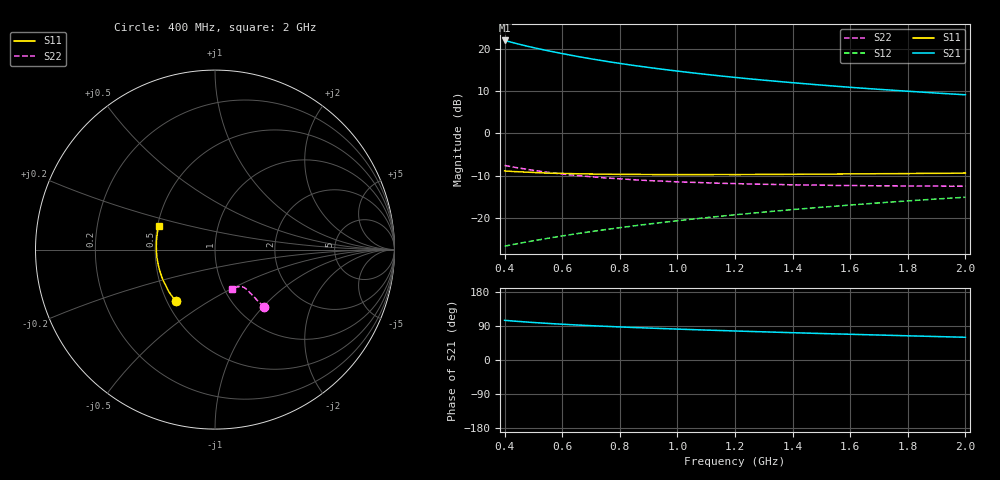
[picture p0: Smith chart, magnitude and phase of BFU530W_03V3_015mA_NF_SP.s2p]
! Filename:  P:\Prog\Test\Noise\ATS_data\Testdata_Net\06 Compressed Noise after Statistics\BFU530W_APM2013_09_A05_03p3V_015mA_NF_CM01_D.sf
! Date/Time: Tue 26/Mar/2013 18:06:07
! BFU530W_APM2013_09_A05_03p3V_1to25mA_NF_CM01_Bias7_R.sf
! Noise Parameter Data File
! BFU530W_APM2013_09_A05_03p3V_1to25mA_NF_CM01
! Date/time: Thu Mar 21 19:18:02 2013
! VAR V_out= 3.300000
! VAR I_out= 14.990000
! VAR V_in= 0.842700
! VAR I_in= 0.164000
! Device data file deembeded for feedlines and parallel
! Original file: \06 Compressed Noise after Statistics\BFU530W_APM2013_09_A05_03p3V_015mA_NF_CM01_R.sf
! Feed-files: PR019V01_070313_Feed1.s2p, PR019V01_070313_Feed2.s2p
! Parallel-file: PR019V01_070313_Par.s2p
# MHz S MA R 50
!  Freq-MHz  S11-mag  S11-arg  S21-mag  S21-arg  S12-mag  S12-arg  S22-mag  S22-arg
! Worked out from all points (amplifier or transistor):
!   37 points, 400 MHz to 2 GHz, reference 50 ohm
!   highest |S21| = 22.0 dB at 400 MHz (marker M1)
!   |S21| within 3 dB of that: start of sweep to 592 MHz
!   unconditionally stable (mu >= 1): 1.143 GHz to end of sweep
!   at 500 MHz: K = 0.84, MSG = 22.9 dB, |S12| = -25.4 dB
!   at 1.1 GHz: K = 1.00, MSG = 17.0 dB, |S12| = -19.9 dB
!   at 2 GHz: K = 1.01, MAG = 11.5 dB, |S12| = -15.1 dB
!   lowest NFmin = 0.87 dB at 420 MHz
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400  0.3599 -127.5  12.64 104.7  0.04629 62.8  0.4188 -49.3
420  0.3567 -130.3  12.12 103.4  0.04779 63.0  0.4065 -49.6
433  0.3538 -131.9  11.81 102.7  0.04871 63.2  0.3988 -49.8
460  0.3507 -135.1  11.2 101.1  0.05069 63.5  0.3851 -50.0
500  0.3454 -139.6  10.4 99.0  0.0536 64.0  0.366 -50.3
550  0.3389 -144.2  9.557 96.6  0.05734 64.8  0.347 -50.4
600  0.3367 -148.5  8.837 94.4  0.06118 65.3  0.3307 -50.6
650  0.3335 -152.4  8.206 92.4  0.06501 65.8  0.3184 -50.7
700  0.3312 -155.9  7.66 90.6  0.06884 66.2  0.3074 -51.0
750  0.3298 -159.0  7.182 88.9  0.07272 66.7  0.2976 -51.0
800  0.3279 -162.1  6.761 87.3  0.07665 67.0  0.2908 -51.4
850  0.3277 -164.9  6.386 85.7  0.08058 67.3  0.283 -51.6
950  0.3261 -169.7  5.755 82.9  0.0886 67.7  0.2725 -52.2
1050  0.3262 -174.0  5.235 80.2  0.09668 68.0  0.264 -52.8
1150  0.3269 -178.1  4.802 77.8  0.1048 68.1  0.257 -53.7
1200  0.3262 -179.9  4.616 76.6  0.1089 68.1  0.2553 -54.4
1250  0.3268 178.2  4.438 75.4  0.113 68.1  0.2521 -54.8
1350  0.3277 175.1  4.133 73.2  0.1214 68.0  0.2489 -56.0
1500  0.3298 170.3  3.744 69.9  0.1338 67.6  0.2446 -58.2
1650  0.3325 166.0  3.425 66.9  0.1464 67.2  0.241 -60.2
1750  0.3343 163.5  3.249 64.9  0.1548 66.8  0.24 -61.7
2000  0.3405 157.2  2.874 60.0  0.1759 65.6  0.238 -66.2
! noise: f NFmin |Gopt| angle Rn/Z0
400  0.8892  0.2  -170.9  0.0742
460  0.8851  0.2294  -176.6  0.067
600  0.8926  0.2244  -173.6  0.07
800  0.94  0.2438  -170.1  0.0675
1000  0.9572  0.2599  -166.8  0.0668
1200  0.9996  0.2575  -162.6  0.0719
1400  0.9929  0.2882  -159.5  0.0701
1600  1.003  0.2949  -157.2  0.0733
1800  1.046  0.3058  -152.6  0.0762
2000  1.094  0.3182  -149.3  0.0827
